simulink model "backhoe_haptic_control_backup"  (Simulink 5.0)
settings: Solver=ode5  StartTime=0.0  StopTime=inf  FixedStep=0.001  RelTol=1e-3
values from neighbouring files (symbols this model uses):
  a1 = 8.5    [startup.m]
  a2 = 48    [startup.m]
  a3 = 38+11/16    (= 38.6875)    [startup.m]
  a4 = 18.5    [startup.m]
  Butter_Order = 2    [startup.m]
  c1 = [-0.0009634 -0.4050766 2.3355377]    [startup.m]
  c2 = [ -0.00644514 2.23812750 22.79925627]    [startup.m]
  c3 = [-0.0057802 2.2376391 22.8266324]    [startup.m]
  c4 = [-0.0020828 1.5286223 20.3434998]    [startup.m]
  R1A = 10    [startup.m]
  R1B = 35.875    [startup.m]
  R2C = 36    [startup.m]
  R2D = 9+7/8    (= 9.875)    [startup.m]
  R3F = 4.5    [startup.m]
  R3G = 5.5    [startup.m]
  REF = 29.625    [startup.m]
  RFH = 9.5    [startup.m]
  RGH = 9.5    [startup.m]
  T01A = acos(RAJ/R1A)    [startup.m]
  T12C = acos((a2^2 + R2C^2 - R1C^2)/(2*a2*R2C))    [startup.m]
  T23D = 0.1317    [startup.m]
  TB12 = acos((R1B^2 + a2^2 - R2B^2)/(2*a2*R1B))    [startup.m]
  TD23 = acos((R2D^2 + a3^2 - R3D^2)/(2*a3*R2D))    [startup.m]
  TDFE = 0.0503    [startup.m]
  TG34 = 1.6966    [startup.m]
undefined symbols (not defined in the file or in its folder): channels, com, ended, Single, uint
libraries: dsparch4 x18, xpclib x8, simulink x1

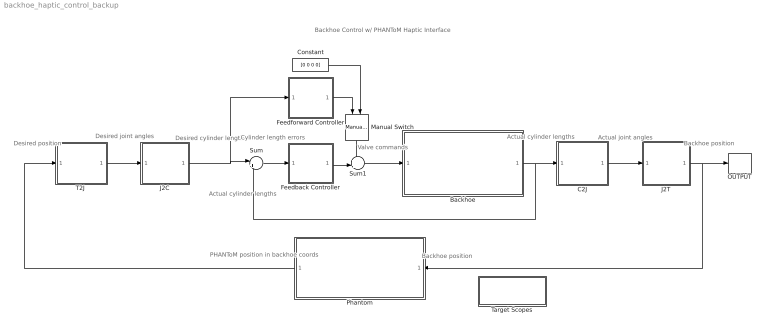
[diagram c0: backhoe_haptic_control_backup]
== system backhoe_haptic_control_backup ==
  note: Desired cylinder lengths
  note: Cylinder length errors
  note: Actual cylinder lengths
  note: Actual cylinder lengths
  note: Backhoe position
  note: Backhoe position
  note: PHANToM position in backhoe coords
  note: Desired joint angles
  note: Desired position
  note: Backhoe Control w/ PHANToM Haptic Interface
  note: Actual joint angles
  note: Valve commands
  Backhoe : Subsystem
  C2J : Subsystem
  Constant : Constant  Value=[0 0 0 0]
  Feedback Controller : Subsystem
  Feedforward Controller : Subsystem
  J2C : Subsystem
  J2T : Subsystem
  Manual Switch : simulink/Signal Routing/Manual Switch  Orientation=down  sw=0  action=0
  OUTPUT : ToWorkspace  VariableName=yb  SampleTime=-1  SaveFormat=StructureWithTime
  Phantom : Subsystem  Orientation=left
  Sum : Sum  Inputs=|+-
  Sum1 : Sum  Inputs=++|
  "T2J " : Subsystem
  Target Scopes : Subsystem
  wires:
  Sum/1 -> Feedback Controller/1(e)
  Backhoe/1(yc) -> Sum/2, C2J/1(yc)
  "T2J "/1(qdes) -> J2C/1(qdes)
  Feedback Controller/1(Us) -> Sum1/2
  Sum1/1 -> Backhoe/1(Us)
  Phantom/1(Yb_Desired) -> "T2J "/1(yp)
  J2C/1(ycdes) -> Sum/1, Feedforward Controller/1(ycdes)
  Manual Switch/1 -> Sum1/1
  Feedforward Controller/1(UsFF) -> Manual Switch/1
  Constant/1 -> Manual Switch/2
  C2J/1(q) -> J2T/1(q)
  J2T/1(yb) -> OUTPUT/1, Phantom/1(Yb)

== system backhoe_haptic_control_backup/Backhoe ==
  note: Valve commands
  note: Position sensor signals
  note: Cylinder lengths
  note: Pressure sensor signals
  Us : Inport
  Anti-Deadband Block : Subsystem
  Backhoe Interface : Subsystem
  Position sensor conversions : Subsystem
  T : Terminator
  yc : Outport
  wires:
  Backhoe Interface/1(Vpos) -> Position sensor conversions/1(Vc)
  Position sensor conversions/1(yc) -> yc/1
  Us/1 -> Anti-Deadband Block/1(us)
  Backhoe Interface/2(Vpres) -> T/1
  Anti-Deadband Block/1(Us) -> Backhoe Interface/1(Us)

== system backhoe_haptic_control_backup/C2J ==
  note: Swing
  note: q1
  note: Cylinder to Joint Transformation
  yc : Inport
  Boom : Subsystem
  Bucket : Subsystem
  Demux : Demux
  Mux : Mux
  Stick : Subsystem
  q : Outport
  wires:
  Mux/1 -> q/1, [GLOBAL_q]
  yc/1 -> Demux/1
  Boom/1(q2) -> Mux/2
  Demux/2 -> Boom/1(yc3)
  Demux/1 -> Mux/1
  Demux/3 -> Stick/1(yc4)
  Stick/1(q3) -> Mux/3
  Demux/4 -> Bucket/1(yc5)
  Bucket/1(q4) -> Mux/4

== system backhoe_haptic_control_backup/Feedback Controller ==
  e : Inport
  Demux : Demux
  Mux : Mux
  "boom [in/s] -> [V]" : Lookup  InputValues=[-1 0 1]  OutputValues=[-0.05 0 0.6]  ShowAdditionalParam=on
  "bucket [in/s] -> [V]" : Lookup  InputValues=[-1 0 1]  OutputValues=[-0.2 0 0.2]  ShowAdditionalParam=on
  "stick [in/s] -> [V]" : Lookup  InputValues=[-1 0 1]  OutputValues=[-0.2 0 0.2]  ShowAdditionalParam=on
  "swing [rad/s] -> [V]" : Lookup  InputValues=[-1 0 1]  OutputValues=[-0.2 0 0.2]  ShowAdditionalParam=on
  Us : Outport
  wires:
  e/1 -> [GLOBAL_e], Demux/1
  Demux/1 -> "swing [rad/s] -> [V]"/1
  "swing [rad/s] -> [V]"/1 -> Mux/1
  Demux/2 -> "boom [in/s] -> [V]"/1
  "boom [in/s] -> [V]"/1 -> Mux/2
  Demux/3 -> "stick [in/s] -> [V]"/1
  "stick [in/s] -> [V]"/1 -> Mux/3
  Demux/4 -> "bucket [in/s] -> [V]"/1
  "bucket [in/s] -> [V]"/1 -> Mux/4
  Mux/1 -> Us/1

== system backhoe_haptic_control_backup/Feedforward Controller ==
  note: This block uses empirical data from the open-loop velocity response to a constant voltage command to the valves. Relationships have been inverted to determine the required voltage to produce a desired velocity for each function.
  note: Feedforward Controller
  ycdes : Inport
  Demux : Demux
  Derivative : Derivative
  Filters : Subsystem
  Gain : Gain  Gain=1/3
  Mux : Mux
  "boom [in/s] -> [V]" : Lookup  InputValues=[-1.0 0 3.0]  OutputValues=[-0.25 0 0.25]  ShowAdditionalParam=on
  "bucket [in/s] -> [V]" : Lookup  InputValues=[-2.3 0 2.75]  OutputValues=[-0.25 0 0.25]  ShowAdditionalParam=on
  "stick [in/s] -> [V]" : Lookup  InputValues=[-1.6 0 1.75]  OutputValues=[-0.25 0 0.25]  ShowAdditionalParam=on
  "swing [rad/s] -> [V]" : Lookup  InputValues=[-0.6 0 0.7]  OutputValues=[-0.25 0 0.25]  ShowAdditionalParam=on
  UsFF : Outport
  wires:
  ycdes/1 -> Filters/1(unfiltered)
  Derivative/1 -> Demux/1
  Demux/1 -> "swing [rad/s] -> [V]"/1
  "swing [rad/s] -> [V]"/1 -> Mux/1
  Demux/2 -> "boom [in/s] -> [V]"/1
  "boom [in/s] -> [V]"/1 -> Mux/2
  Demux/3 -> "stick [in/s] -> [V]"/1
  "stick [in/s] -> [V]"/1 -> Mux/3
  Demux/4 -> "bucket [in/s] -> [V]"/1
  "bucket [in/s] -> [V]"/1 -> Mux/4
  Mux/1 -> Gain/1
  Filters/1(filtered) -> Derivative/1
  Gain/1 -> UsFF/1

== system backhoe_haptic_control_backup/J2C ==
  note: Joint Space -> Cylinder Space Transformation
  note: Swing Cylinders
  qdes : Inport
  Boom cylinder : Subsystem
  Bucket cylinder : Subsystem
  Demux : Demux
  Mux : Mux
  Stick cylinder : Subsystem
  overswing  protection : Saturate  UpperLimit=pi/3  LowerLimit=-pi/2
  ycdes : Outport
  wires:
  qdes/1 -> Demux/1
  Mux/1 -> ycdes/1
  Demux/2 -> Boom cylinder/1(q2)
  Boom cylinder/1(yc3) -> Mux/2
  Demux/3 -> Stick cylinder/1(q3)
  Stick cylinder/1(yc4) -> Mux/3
  Demux/4 -> Bucket cylinder/1(q4)
  Bucket cylinder/1(yc5) -> Mux/4
  Demux/1 -> overswing  protection/1
  overswing  protection/1 -> Mux/1

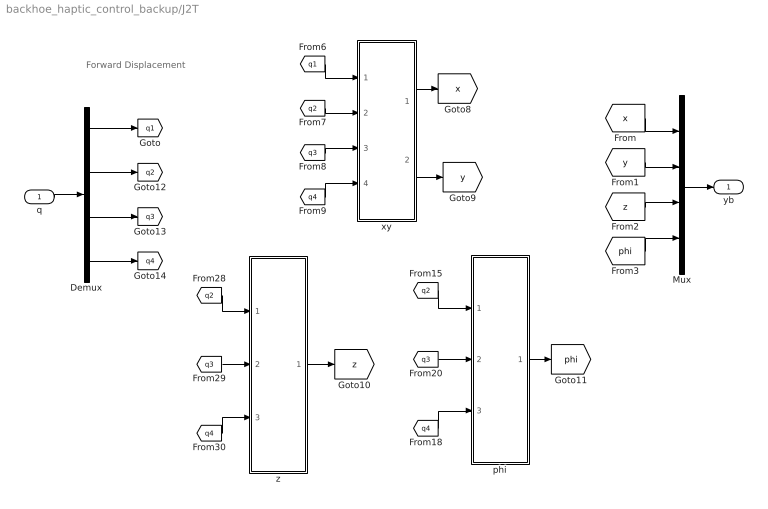
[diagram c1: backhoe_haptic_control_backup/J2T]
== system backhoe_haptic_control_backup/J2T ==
  note: Forward Displacement
  q : Inport
  Demux : Demux
  Mux : Mux
  phi : Subsystem
  xy : Subsystem
  z : Subsystem
  yb : Outport
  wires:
  [q2] -> z/1(q2)
  [q3] -> z/2(q3)
  [q4] -> z/3(q4)
  z/1(z) -> [z]
  q/1 -> Demux/1
  Demux/2 -> [q2]
  Demux/1 -> [q1]
  Demux/3 -> [q3]
  Demux/4 -> [q4]
  [q2] -> phi/1(q2)
  [q3] -> phi/2(q3)
  phi/1(phi) -> [phi]
  Mux/1 -> yb/1
  [x] -> Mux/1
  [y] -> Mux/2
  [z] -> Mux/3
  [phi] -> Mux/4
  xy/1(x) -> [x]
  [q1] -> xy/1(q1)
  [q2] -> xy/2(q2)
  [q3] -> xy/3(q3)
  [q4] -> xy/4(q4)
  [q4] -> phi/3(q4)
  xy/2(y) -> [y]

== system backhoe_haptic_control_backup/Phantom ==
  Yb : Inport
  Phantom Interface : Subsystem
  Supervisory Control : Subsystem
  Yb_Desired : Outport
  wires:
  Yb/1 -> Supervisory Control/1(Y_Bh)
  Supervisory Control/1(Y_Bh_ref) -> Yb_Desired/1, [GLOBAL_YB_DES]
  Phantom Interface/2(Ph_Time) -> Supervisory Control/3(Ph_Time)
  Phantom Interface/3(Ph_Flag) -> Supervisory Control/4(Ph Flag)
  Supervisory Control/3(OUt_Flag) -> Phantom Interface/2(Bh_Flag)
  Supervisory Control/2(Send2Ph) -> Phantom Interface/1(Yb)
  Phantom Interface/1("Yp ") -> Supervisory Control/2(Y_Ph_In)

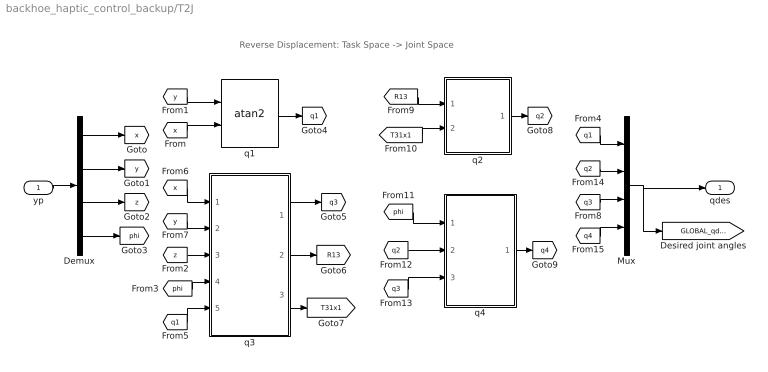
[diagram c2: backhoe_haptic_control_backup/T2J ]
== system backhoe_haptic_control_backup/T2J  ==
  note: Reverse Displacement: Task Space -> Joint Space
  yp : Inport
  Demux : Demux
  Mux : Mux
  q1 : Trigonometry  Operator=atan2
  q2 : Subsystem
  q3 : Subsystem
  q4 : Subsystem
  qdes : Outport
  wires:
  [x] -> q3/1(x)
  [y] -> q3/2(y)
  [z] -> q3/3(z)
  [phi] -> q3/4(phi)
  [q1] -> q3/5(q1)
  q3/1(q3) -> [q3]
  q3/2(R13) -> [R13]
  [y] -> q1/1
  [x] -> q1/2
  q1/1 -> [q1]
  q3/3(T31x1) -> [T31x1]
  [R13] -> q2/1(R13)
  [T31x1] -> q2/2(T31x1)
  [q3] -> q4/3(q3)
  [q2] -> q4/2(q2)
  [phi] -> q4/1(phi)
  q2/1(q2) -> [q2]
  q4/1(q4) -> [q4]
  Mux/1 -> qdes/1, [GLOBAL_qdes]
  [q1] -> Mux/1
  [q3] -> Mux/3
  [q2] -> Mux/2
  [q4] -> Mux/4
  yp/1 -> Demux/1
  Demux/1 -> [x]
  Demux/2 -> [y]
  Demux/3 -> [z]
  Demux/4 -> [phi]

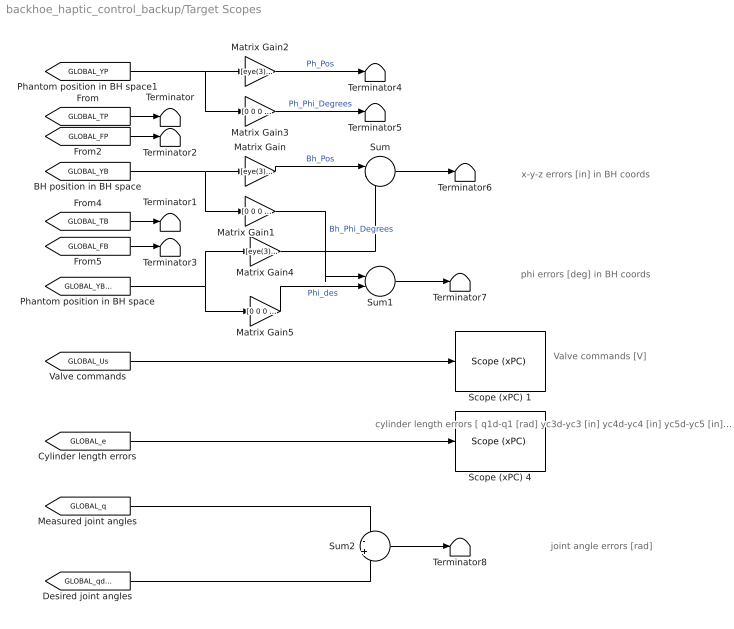
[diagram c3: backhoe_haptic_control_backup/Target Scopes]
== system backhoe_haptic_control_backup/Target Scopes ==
  note: x-y-z errors [in] in BH coords
  note: phi errors [deg] in BH coords
  note: Valve commands [V]
  note: cylinder length errors [ q1d-q1 [rad] yc3d-yc3 [in] yc4d-yc4 [in] yc5d-yc5 [in] ]
  note: joint angle errors [rad]
  Matrix Gain : Gain  Gain=[eye(3) zeros(3,1)]  Multiplication=Matrix(K*u)
  Matrix Gain1 : Gain  Gain=[0 0 0 180/pi]  Multiplication=Matrix(K*u)
  Matrix Gain2 : Gain  Gain=[eye(3) zeros(3,1)]  Multiplication=Matrix(K*u)
  Matrix Gain3 : Gain  Gain=[0 0 0 180/pi]  Multiplication=Matrix(K*u)
  Matrix Gain4 : Gain  Gain=[eye(3) zeros(3,1)]  Multiplication=Matrix(K*u)
  Matrix Gain5 : Gain  Gain=[0 0 0 180/pi]  Multiplication=Matrix(K*u)
  Scope (xPC) 1 : xpclib/Misc./Scope (xPC)   scopeno=3  scopetype=Target  viewmode=Graphical redraw  grid=on  ylimits=[0,12]  autostart=on  nosamples=1000  noprepostsamples=0  interleave=1  triggermode=FreeRun  triggersignal=1  triggerlevel=0.0  triggerslope=either  triggerscope=1  triggersample=0
  Scope (xPC) 4 : xpclib/Misc./Scope (xPC)   scopeno=4  scopetype=Target  viewmode=Graphical redraw  grid=on  ylimits=[-5,5]  autostart=on  nosamples=1000  noprepostsamples=0  interleave=1  triggermode=FreeRun  triggersignal=1  triggerlevel=0.0  triggerslope=either  triggerscope=1  triggersample=0
  Sum : Sum  Inputs=|-+
  Sum1 : Sum  Inputs=|-+
  Sum2 : Sum  Inputs=-+
  Terminator{,1..8} (9 alike) : Terminator
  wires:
  [GLOBAL_TP] -> Terminator/1
  [GLOBAL_TB] -> Terminator1/1
  [GLOBAL_YB] -> Matrix Gain/1, Matrix Gain1/1
  [GLOBAL_YP] -> Matrix Gain2/1, Matrix Gain3/1
  [GLOBAL_FP] -> Terminator2/1
  [GLOBAL_FB] -> Terminator3/1
  Sum1/1 -> Terminator7/1
  Matrix Gain5/1 -> Sum1/2  "Phi_des"
  Matrix Gain1/1 -> Sum1/1  "Bh_Phi_Degrees"
  Sum/1 -> Terminator6/1
  Matrix Gain/1 -> Sum/1  "Bh_Pos"
  Matrix Gain4/1 -> Sum/2
  Matrix Gain2/1 -> Terminator4/1  "Ph_Pos"
  Matrix Gain3/1 -> Terminator5/1  "Ph_Phi_Degrees"
  [GLOBAL_Us] -> Scope (xPC) 1/1
  Sum2/1 -> Terminator8/1
  [GLOBAL_YB_DES] -> Matrix Gain4/1, Matrix Gain5/1
  [GLOBAL_e] -> Scope (xPC) 4/1
  [GLOBAL_q] -> Sum2/1
  [GLOBAL_qdes] -> Sum2/2

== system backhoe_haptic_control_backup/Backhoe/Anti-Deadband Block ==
  note: This block take a servo commmand that saturates at +-1 and converts it into valve signals. "u" in the input signal which a 4-vector. Neutral is half the voltage supplied Vc to the valves which should 6V = 1/2 * 12V. Commands to the valve must be between 25% AND 75% of Vc where 50% is neutral or the "zero command" that tell the valve to stop flow to the valve. Neutral can either be set at 6V of measure from Channel 15.
  us : Inport
  Demux : Demux
  Look-Up Table{,1..3} (4 alike) : Lookup  InputValues=[-1 -0.02 0.02 1]  OutputValues=[3 5.45 6.55 9]  ShowAdditionalParam=on  LookUpMeth=Interpolation-Use End Values  OutDataTypeMode=double
  Mux : Mux
  Us : Outport
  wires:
  Look-Up Table/1 -> Mux/1
  Look-Up Table1/1 -> Mux/2
  Demux/1 -> Look-Up Table/1
  Demux/2 -> Look-Up Table1/1
  Demux/3 -> Look-Up Table2/1
  Look-Up Table2/1 -> Mux/3
  Demux/4 -> Look-Up Table3/1
  Look-Up Table3/1 -> Mux/4
  Mux/1 -> Us/1
  us/1 -> Demux/1

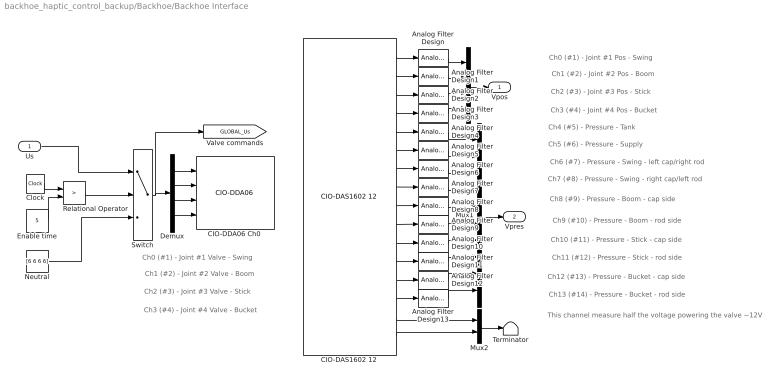
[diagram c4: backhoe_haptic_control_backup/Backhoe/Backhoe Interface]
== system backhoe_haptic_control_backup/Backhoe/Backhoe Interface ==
  note: Ch0 (#1) - Joint #1 Valve - Swing
  note: Ch1 (#2) - Joint #2 Valve - Boom
  note: Ch2 (#3) - Joint #3 Valve - Stick
  note: Ch3 (#4) - Joint #4 Valve - Bucket
  note: Ch0 (#1) - Joint #1 Pos - Swing
  note: Ch1 (#2) - Joint #2 Pos - Boom
  note: Ch2 (#3) - Joint #3 Pos - Stick
  note: Ch3 (#4) - Joint #4 Pos - Bucket
  note: Ch4 (#5) - Pressure - Tank
  note: Ch5 (#6) - Pressure - Supply
  note: Ch6 (#7) - Pressure - Swing - left cap/right rod
  note: Ch7 (#8) - Pressure - Swing - right cap/left rod
  note: Ch8 (#9) - Pressure - Boom - cap side
  note: Ch9 (#10) - Pressure - Boom - rod side
  note: Ch10 (#11) - Pressure - Stick - cap side
  note: Ch11 (#12) - Pressure - Stick - rod side
  note: Ch12 (#13) - Pressure - Bucket - cap side
  note: Ch13 (#14) - Pressure - Bucket - rod side
  note: This channel measure half the voltage powering the valve ~12V
  Us : Inport
  Analog Filter Design{,1..13} (14 alike) : dsparch4/Analog Filter Design  method=Butterworth  filttype=Lowpass  N=Butter_Order  Wlo=Butter_Rad  Whi=80  Rp=2  Rs=40
  "CIO-DAS1602 12 " : xpclib/A//D/Computer Boards/CIO-DAS1602 12   channel=16  range=0-10V  mux=Single-ended (16 channels)  sampletime=0.001  baseaddress=0x340
  "CIO-DDA06 Ch0 " : xpclib/D//A/Computer Boards/CIO-DDA06   channel=[1 2 3 4]  range=[10 10 10 10]  reset=[1 1 1 1]  initValue=[6 6 6 6]  sampletime=0.001  baseaddress=0x300
  Clock : Clock
  Demux : Demux
  Enable time : Constant  Value=5
  Mux : Mux
  Mux1 : Mux  Inputs=10
  Mux2 : Mux  Inputs=2
  Neutral : Constant  Value=[6 6 6 6]  ShowAdditionalParam=on
  Relational Operator : RelationalOperator  Operator=>  ShowAdditionalParam=on
  Switch : Switch  Threshold=0.5  ShowAdditionalParam=on
  Terminator : Terminator
  Vpos : Outport
  Vpres : Outport  Port=2
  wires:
  Demux/1 -> "CIO-DDA06 Ch0 "/1
  Demux/2 -> "CIO-DDA06 Ch0 "/2
  Demux/3 -> "CIO-DDA06 Ch0 "/3
  Demux/4 -> "CIO-DDA06 Ch0 "/4
  Mux/1 -> Vpos/1
  "CIO-DAS1602 12 "/1 -> Analog Filter Design/1
  Analog Filter Design/1 -> Mux/1
  "CIO-DAS1602 12 "/2 -> Analog Filter Design1/1
  "CIO-DAS1602 12 "/3 -> Analog Filter Design2/1
  "CIO-DAS1602 12 "/4 -> Analog Filter Design3/1
  Analog Filter Design1/1 -> Mux/2
  Analog Filter Design2/1 -> Mux/3
  Analog Filter Design3/1 -> Mux/4
  "CIO-DAS1602 12 "/5 -> Analog Filter Design4/1
  "CIO-DAS1602 12 "/6 -> Analog Filter Design5/1
  "CIO-DAS1602 12 "/7 -> Analog Filter Design6/1
  "CIO-DAS1602 12 "/8 -> Analog Filter Design7/1
  "CIO-DAS1602 12 "/9 -> Analog Filter Design8/1
  "CIO-DAS1602 12 "/10 -> Analog Filter Design9/1
  "CIO-DAS1602 12 "/11 -> Analog Filter Design10/1
  "CIO-DAS1602 12 "/12 -> Analog Filter Design11/1
  "CIO-DAS1602 12 "/13 -> Analog Filter Design12/1
  "CIO-DAS1602 12 "/14 -> Analog Filter Design13/1
  "CIO-DAS1602 12 "/15 -> Mux2/1
  Analog Filter Design4/1 -> Mux1/1
  Analog Filter Design5/1 -> Mux1/2
  Analog Filter Design6/1 -> Mux1/3
  Analog Filter Design7/1 -> Mux1/4
  Analog Filter Design8/1 -> Mux1/5
  Analog Filter Design9/1 -> Mux1/6
  Analog Filter Design10/1 -> Mux1/7
  Analog Filter Design11/1 -> Mux1/8
  Analog Filter Design12/1 -> Mux1/9
  Analog Filter Design13/1 -> Mux1/10
  Mux1/1 -> Vpres/1
  Mux2/1 -> Terminator/1
  "CIO-DAS1602 12 "/16 -> Mux2/2
  Switch/1 -> Demux/1, [GLOBAL_Us]
  Clock/1 -> Relational Operator/1
  Enable time/1 -> Relational Operator/2
  Relational Operator/1 -> Switch/2
  Neutral/1 -> Switch/3
  Us/1 -> Switch/1

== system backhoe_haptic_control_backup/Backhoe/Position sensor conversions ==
  note: Sensor Conversions
  Vc : Inport
  Boom sensor : Subsystem
  Bucket sensor : Subsystem
  Demux : Demux
  Mux : Mux
  Stick sensor : Subsystem
  Swing pot : Subsystem
  yc : Outport
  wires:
  Vc/1 -> Demux/1
  Demux/1 -> Swing pot/1(Vc1)
  Demux/2 -> Boom sensor/1(Vc2)
  Swing pot/1(q1) -> Mux/1
  Boom sensor/1(yc3) -> Mux/2
  Demux/3 -> Stick sensor/1(Vc3)
  Stick sensor/1(yc4) -> Mux/3
  Mux/1 -> yc/1
  Demux/4 -> Bucket sensor/1(Vc4)
  Bucket sensor/1(yc5) -> Mux/4

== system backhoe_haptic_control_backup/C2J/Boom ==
  note: TA1B
  yc3 : Inport
  CosineLawA : Subsystem
  R1A : Constant  Value=R1A
  R1B : Constant  Value=R1B
  Sum : Sum  Inputs=+---
  T01A : Constant  Value=T01A
  TA1B : Constant  Value=TB12
  pi : Constant  Value=pi
  q2 : Outport
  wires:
  pi/1 -> Sum/1
  T01A/1 -> Sum/2
  TA1B/1 -> Sum/4
  CosineLawA/1(theta) -> Sum/3
  R1A/1 -> CosineLawA/1(r1)
  R1B/1 -> CosineLawA/2(r2)
  Sum/1 -> q2/1
  yc3/1 -> CosineLawA/3(r3)

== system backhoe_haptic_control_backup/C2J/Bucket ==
  yc5 : Inport
  R3F : Constant  Value=R3F
  R3G : Constant  Value=R3G
  R3H : Subsystem
  REF : Constant  Value=REF
  RFH : Constant  Value=RFH
  RGH : Constant  Value=RGH
  Sum : Sum  Inputs=+----
  T23D : Constant  Value=T23D
  TEFH : Subsystem
  TF3H : Subsystem
  TG34 : Constant  Value=TG34
  TH3G : Subsystem
  THF3 : Subsystem
  pi : Constant  Value=3*pi
  q4 : Outport
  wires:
  TEFH/1(TEFH) -> THF3/1(TEFH)
  REF/1 -> TEFH/1(r1)
  yc5/1 -> TEFH/3(r3)
  RFH/1 -> TEFH/2(r2), R3H/2(RFH), TF3H/3(r3)
  THF3/1(THF3) -> R3H/1(THF3)
  R3F/1 -> TF3H/1(r1)
  R3H/1(R3H) -> TF3H/2(r2), TH3G/1(r1)
  R3G/1 -> TH3G/2(r2)
  RGH/1 -> TH3G/3(r3)
  pi/1 -> Sum/1
  Sum/1 -> q4/1
  T23D/1 -> Sum/5
  TG34/1 -> Sum/4
  TH3G/1(TH3G) -> Sum/2
  TF3H/1(TF3H) -> Sum/3

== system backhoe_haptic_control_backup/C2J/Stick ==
  note: TC2D
  yc4 : Inport
  CosineLawA : Subsystem
  R2C : Constant  Value=R2C
  R2D : Constant  Value=R2D
  Sum : Sum  Inputs=+---
  T12C : Constant  Value=T12C
  TD23 : Constant  Value=TD23
  pi : Constant  Value=3*pi
  q3 : Outport
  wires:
  pi/1 -> Sum/1
  T12C/1 -> Sum/2
  TD23/1 -> Sum/4
  CosineLawA/1(theta) -> Sum/3
  R2C/1 -> CosineLawA/1(r1)
  R2D/1 -> CosineLawA/2(r2)
  Sum/1 -> q3/1
  yc4/1 -> CosineLawA/3(r3)

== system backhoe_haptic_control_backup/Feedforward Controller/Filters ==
  unfiltered : Inport
  Analog Filter Design{,1..3} (4 alike) : dsparch4/Analog Filter Design  method=Butterworth  filttype=Lowpass  N=2  Wlo=2*pi*5  Whi=80  Rp=2  Rs=40
  Demux : Demux
  Mux : Mux
  filtered : Outport
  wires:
  unfiltered/1 -> Demux/1
  Demux/1 -> Analog Filter Design/1
  Analog Filter Design/1 -> Mux/1
  Demux/2 -> Analog Filter Design1/1
  Analog Filter Design1/1 -> Mux/2
  Demux/3 -> Analog Filter Design2/1
  Analog Filter Design2/1 -> Mux/3
  Demux/4 -> Analog Filter Design3/1
  Analog Filter Design3/1 -> Mux/4
  Mux/1 -> filtered/1

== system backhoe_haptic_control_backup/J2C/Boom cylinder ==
  q2 : Inport
  Constant : Constant  Value=pi
  Constant1 : Constant  Value=T01A
  Constant2 : Constant  Value=TB12
  CosineLawB : Subsystem
  Sum : Sum  Inputs=+---
  yc3 : Outport
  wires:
  Constant/1 -> Sum/1
  Constant1/1 -> Sum/2
  Sum/1 -> CosineLawB/1(TA1B)
  CosineLawB/1(yc3) -> yc3/1
  q2/1 -> Sum/3
  Constant2/1 -> Sum/4

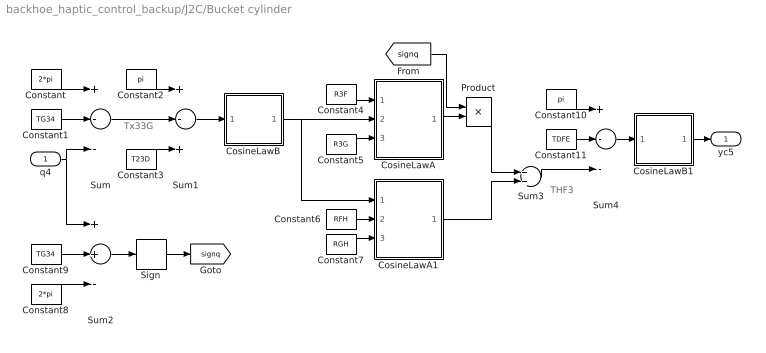
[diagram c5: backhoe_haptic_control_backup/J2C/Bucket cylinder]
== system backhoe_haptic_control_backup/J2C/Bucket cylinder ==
  note: Tx33G
  note: THF3
  q4 : Inport
  Constant : Constant  Value=2*pi
  Constant1 : Constant  Value=TG34
  Constant10 : Constant  Value=pi
  Constant11 : Constant  Value=TDFE
  Constant2 : Constant  Value=pi
  Constant3 : Constant  Value=T23D
  Constant4 : Constant  Value=R3F
  Constant5 : Constant  Value=R3G
  Constant6 : Constant  Value=RFH
  Constant7 : Constant  Value=RGH
  Constant8 : Constant  Value=2*pi
  Constant9 : Constant  Value=TG34
  CosineLawA : Subsystem
  CosineLawA1 : Subsystem
  CosineLawB : Subsystem
  CosineLawB1 : Subsystem
  Product : Product
  Sign : Signum
  Sum : Sum  Inputs=+--
  Sum1 : Sum  Inputs=+-+
  Sum2 : Sum  Inputs=++-
  Sum3 : Sum
  Sum4 : Sum  Inputs=+--
  yc5 : Outport
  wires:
  Constant/1 -> Sum/1
  Constant1/1 -> Sum/2
  Sum/1 -> Sum1/2
  Constant2/1 -> Sum1/1
  Constant3/1 -> Sum1/3
  Sum1/1 -> CosineLawB/1(TG3F)
  CosineLawB/1(rFG) -> CosineLawA/2(r2), CosineLawA1/1(r1)
  Constant4/1 -> CosineLawA/1(r1)
  Constant5/1 -> CosineLawA/3(r3)
  Constant6/1 -> CosineLawA1/2(r2)
  Constant7/1 -> CosineLawA1/3(r3)
  Constant9/1 -> Sum2/2
  Constant8/1 -> Sum2/3
  Sum2/1 -> Sign/1
  [signq] -> Product/1
  CosineLawA/1(T3FG) -> Product/2
  Sign/1 -> [signq]
  Product/1 -> Sum3/1
  CosineLawA1/1(THFG) -> Sum3/2
  Constant10/1 -> Sum4/1
  Sum3/1 -> Sum4/3
  Constant11/1 -> Sum4/2
  Sum4/1 -> CosineLawB1/1(TEFH)
  CosineLawB1/1(yc5) -> yc5/1
  q4/1 -> Sum/3, Sum2/1

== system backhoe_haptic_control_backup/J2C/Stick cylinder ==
  q3 : Inport
  Constant : Constant  Value=pi
  Constant1 : Constant  Value=TD23
  Constant2 : Constant  Value=T12C
  CosineLawB : Subsystem
  Sum : Sum  Inputs=+---
  yc4 : Outport
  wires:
  Constant/1 -> Sum/1
  Constant1/1 -> Sum/2
  Sum/1 -> CosineLawB/1(TC2D)
  CosineLawB/1(yc4) -> yc4/1
  q3/1 -> Sum/3
  Constant2/1 -> Sum/4

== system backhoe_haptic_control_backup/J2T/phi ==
  q2 : Inport
  q3 : Inport  Port=2
  q4 : Inport  Port=3
  Constant : Constant  Value=3*pi
  Sum : Sum  Inputs=+++-
  phi : Outport
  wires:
  q2/1 -> Sum/1
  q3/1 -> Sum/2
  q4/1 -> Sum/3
  Constant/1 -> Sum/4
  Sum/1 -> phi/1

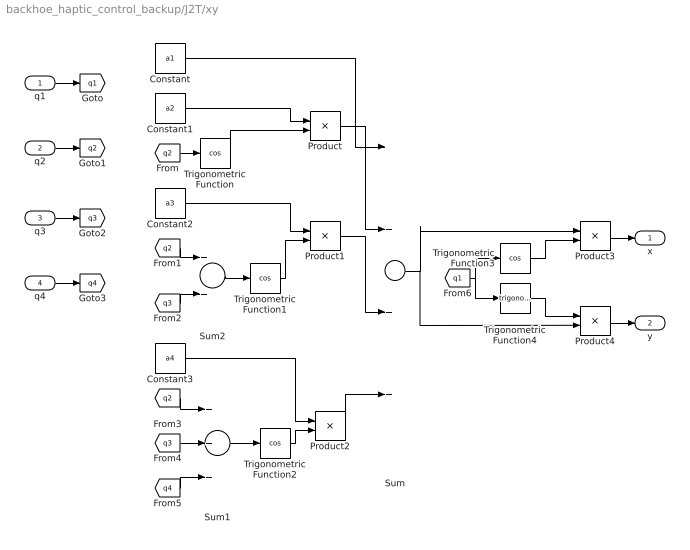
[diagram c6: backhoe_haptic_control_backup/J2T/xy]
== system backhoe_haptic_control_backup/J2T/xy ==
  q1 : Inport
  q2 : Inport  Port=2
  q3 : Inport  Port=3
  q4 : Inport  Port=4
  Constant : Constant  Value=a1
  Constant1 : Constant  Value=a2
  Constant2 : Constant  Value=a3
  Constant3 : Constant  Value=a4
  Product{,1..4} (5 alike) : Product
  Sum : Sum  Inputs=++++
  Sum1 : Sum  Inputs=+++
  Sum2 : Sum
  Trigonometric Function{,1..3} (4 alike) : Trigonometry  Operator=cos
  Trigonometric Function4 : Trigonometry
  x : Outport
  y : Outport  Port=2
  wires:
  q1/1 -> [q1]
  q2/1 -> [q2]
  q3/1 -> [q3]
  q4/1 -> [q4]
  Constant/1 -> Sum/1
  Product/1 -> Sum/2
  Constant1/1 -> Product/1
  [q3] -> Sum2/2
  [q2] -> Sum2/1
  Constant2/1 -> Product1/1
  Product1/1 -> Sum/3
  Product2/1 -> Sum/4
  Constant3/1 -> Product2/1
  [q2] -> Sum1/1
  [q3] -> Sum1/2
  [q4] -> Sum1/3
  Product3/1 -> x/1
  Sum/1 -> Product4/2, Product3/1
  Trigonometric Function/1 -> Product/2
  [q2] -> Trigonometric Function/1
  Sum2/1 -> Trigonometric Function1/1
  Trigonometric Function1/1 -> Product1/2
  Sum1/1 -> Trigonometric Function2/1
  Trigonometric Function2/1 -> Product2/2
  Product4/1 -> y/1
  Trigonometric Function3/1 -> Product3/2
  [q1] -> Trigonometric Function3/1, Trigonometric Function4/1
  Trigonometric Function4/1 -> Product4/1

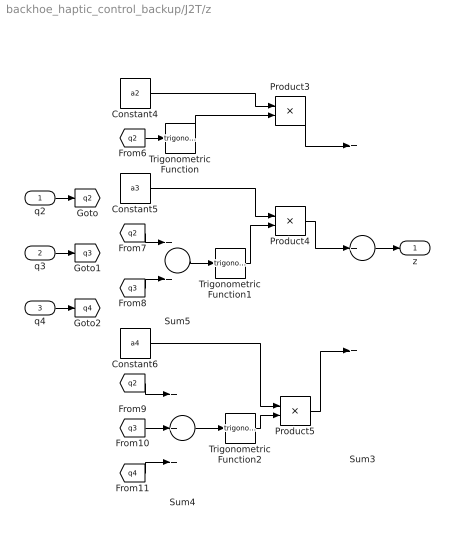
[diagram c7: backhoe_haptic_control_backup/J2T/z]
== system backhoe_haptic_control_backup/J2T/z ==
  q2 : Inport
  q3 : Inport  Port=2
  q4 : Inport  Port=3
  Constant4 : Constant  Value=a2
  Constant5 : Constant  Value=a3
  Constant6 : Constant  Value=a4
  Product3 : Product
  Product4 : Product
  Product5 : Product
  Sum3 : Sum  Inputs=+++
  Sum4 : Sum  Inputs=+++
  Sum5 : Sum
  Trigonometric Function : Trigonometry
  Trigonometric Function1 : Trigonometry
  Trigonometric Function2 : Trigonometry
  z : Outport
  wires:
  q3/1 -> [q3]
  q4/1 -> [q4]
  q2/1 -> [q2]
  Constant4/1 -> Product3/1
  [q3] -> Sum5/2
  [q2] -> Sum5/1
  Constant5/1 -> Product4/1
  Constant6/1 -> Product5/1
  [q2] -> Sum4/1
  [q3] -> Sum4/2
  [q4] -> Sum4/3
  Trigonometric Function/1 -> Product3/2
  [q2] -> Trigonometric Function/1
  Sum5/1 -> Trigonometric Function1/1
  Trigonometric Function1/1 -> Product4/2
  Sum4/1 -> Trigonometric Function2/1
  Trigonometric Function2/1 -> Product5/2
  Product3/1 -> Sum3/1
  Product4/1 -> Sum3/2
  Product5/1 -> Sum3/3
  Sum3/1 -> z/1

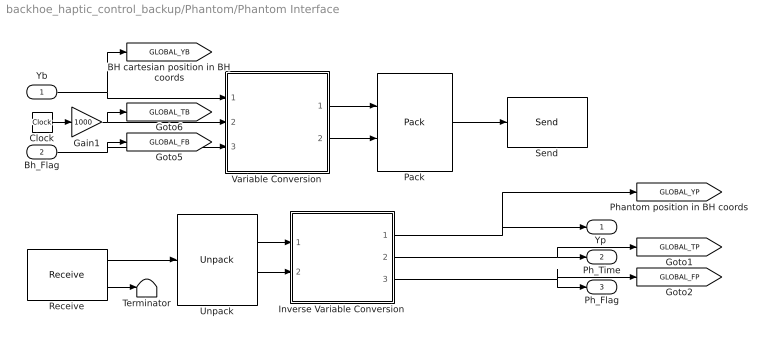
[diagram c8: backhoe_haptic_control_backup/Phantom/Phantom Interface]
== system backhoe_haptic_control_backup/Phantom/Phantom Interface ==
  Yb : Inport
  Bh_Flag : Inport  Port=2
  Clock : Clock
  Gain1 : Gain  Gain=1000  ShowAdditionalParam=on  OutDataTypeMode=Specify via dialog  OutDataType=uint(32)
  Inverse Variable Conversion : Subsystem
  Pack : xpclib/UDP/Pack  datatypes={'double','uint32'}  byteAlign=8
  Receive : xpclib/UDP/Receive  ipAddress=0.0.0.0  ipPort=com.Ph2Bh_Port  width=com.Ph2Bh_Bytes  sampletime=Sampling_Time
  Send : xpclib/UDP/Send  ipAddress=com.SendIP  ipPort=com.Bh2Ph_Port  sampletime=Sampling_Time
  Terminator : Terminator
  Unpack : xpclib/UDP/Unpack  dimensions=com.Ph2Bh_Port_Dim  datatypes={'double','uint32'}  byteAlign=8
  Variable Conversion : Subsystem
  "Yp " : Outport
  Ph_Time : Outport  Port=2
  Ph_Flag : Outport  Port=3
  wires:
  Receive/2 -> Terminator/1
  Receive/1 -> Unpack/1
  Pack/1 -> Send/1
  Yb/1 -> Variable Conversion/1(Yb), [GLOBAL_YB]
  Bh_Flag/1 -> [GLOBAL_FB], Variable Conversion/3(Bh_Flag)
  Unpack/1 -> Inverse Variable Conversion/1(doubles)
  Inverse Variable Conversion/3(Ph_Flag) -> Ph_Flag/1, [GLOBAL_FP]
  Inverse Variable Conversion/2(Ph_Time) -> Ph_Time/1, [GLOBAL_TP]
  Unpack/2 -> Inverse Variable Conversion/2(uint32s)
  Variable Conversion/2(uint32s) -> Pack/2
  Variable Conversion/1(doubles) -> Pack/1
  Clock/1 -> Gain1/1
  Gain1/1 -> [GLOBAL_TB], Variable Conversion/2(Bh_Time)
  Inverse Variable Conversion/1(Yp) -> "Yp "/1, [GLOBAL_YP]

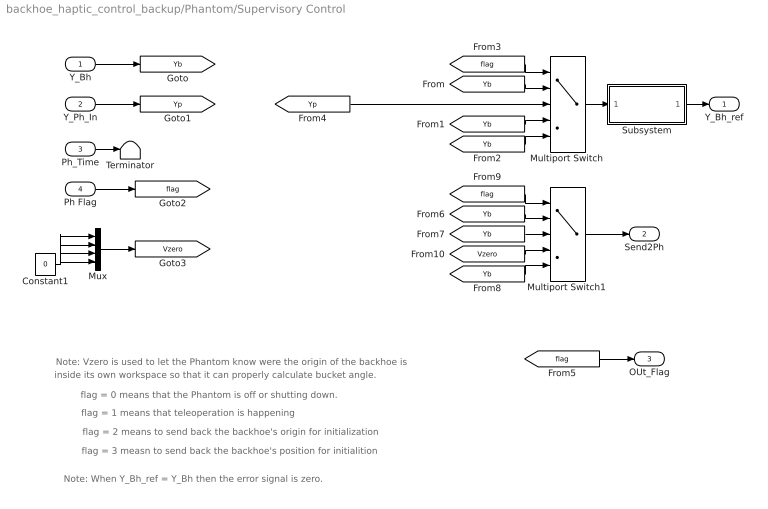
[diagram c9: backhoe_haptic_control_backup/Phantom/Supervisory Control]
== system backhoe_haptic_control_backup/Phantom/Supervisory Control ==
  note: Note: Vzero is used to let the Phantom know were the origin of the backhoe is
  note: flag = 0 means that the Phantom is off or shutting down.
  note: flag = 3 measn to send back the backhoe's position for initialition
  note: inside its own workspace so that it can properly calculate bucket angle.
  note: flag = 1 means that teleoperation is happening
  note: flag = 2 means to send back the backhoe's origin for initialization
  note: Note: When Y_Bh_ref = Y_Bh then the error signal is zero.
  Y_Bh : Inport
  Y_Ph_In : Inport  Port=2
  Ph_Time : Inport  Port=3
  Ph Flag : Inport  Port=4
  Constant1 : Constant  Value=0
  Multiport Switch : MultiPortSwitch  ShowAdditionalParam=on  zeroidx=on
  Multiport Switch1 : MultiPortSwitch  ShowAdditionalParam=on  zeroidx=on
  Mux : Mux
  Subsystem : Subsystem
  Terminator : Terminator
  Y_Bh_ref : Outport
  Send2Ph : Outport  Port=2
  OUt_Flag : Outport  Port=3
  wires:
  Ph_Time/1 -> Terminator/1
  [flag] -> OUt_Flag/1
  Y_Bh/1 -> [Yb]
  Ph Flag/1 -> [flag]
  Constant1/1 -> Mux/1, Mux/4, Mux/3, Mux/2
  Mux/1 -> [Vzero]
  [Yb] -> Multiport Switch/2
  [Yb] -> Multiport Switch/4
  [Yb] -> Multiport Switch/5
  [flag] -> Multiport Switch/1
  [Yb] -> Multiport Switch1/2
  [Vzero] -> Multiport Switch1/4
  [Yb] -> Multiport Switch1/5
  [flag] -> Multiport Switch1/1
  [Yb] -> Multiport Switch1/3
  Multiport Switch1/1 -> Send2Ph/1
  Multiport Switch/1 -> Subsystem/1(Yp)
  Subsystem/1(Y_Bh_REF) -> Y_Bh_ref/1
  [Yp] -> Multiport Switch/3
  Y_Ph_In/1 -> [Yp]

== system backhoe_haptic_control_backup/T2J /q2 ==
  note: T213
  R13 : Inport
  T31x1 : Inport  Port=2
  CosineLawA : Subsystem
  Sum : Sum  Inputs=|++
  a2 : Constant  Value=a2
  a3 : Constant  Value=a3
  q2 : Outport
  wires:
  a2/1 -> CosineLawA/1(r1)
  a3/1 -> CosineLawA/3(r3)
  CosineLawA/1(theta) -> Sum/1
  Sum/1 -> q2/1
  R13/1 -> CosineLawA/2(r2)
  T31x1/1 -> Sum/2

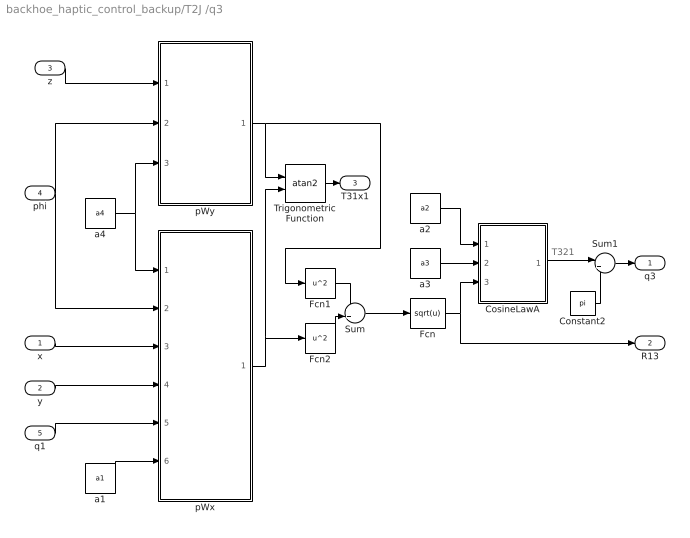
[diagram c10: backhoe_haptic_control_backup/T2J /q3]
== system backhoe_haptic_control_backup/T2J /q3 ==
  note: T321
  x : Inport
  y : Inport  Port=2
  z : Inport  Port=3
  phi : Inport  Port=4
  q1 : Inport  Port=5
  Constant2 : Constant  Value=pi
  CosineLawA : Subsystem
  Fcn : Fcn  Expr=sqrt(u)
  Fcn1 : Fcn  Expr=u^2
  Fcn2 : Fcn  Expr=u^2
  Sum : Sum
  Sum1 : Sum  Inputs=|++
  Trigonometric Function : Trigonometry  Operator=atan2
  a1 : Constant  Value=a1
  a2 : Constant  Value=a2
  a3 : Constant  Value=a3
  a4 : Constant  Value=a4
  pWx : Subsystem
  pWy : Subsystem
  q3 : Outport
  R13 : Outport  Port=2
  T31x1 : Outport  Port=3
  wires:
  a1/1 -> pWx/6(a1)
  q1/1 -> pWx/5(q1)
  y/1 -> pWx/4(y)
  x/1 -> pWx/3(x)
  a4/1 -> pWx/1(a4), pWy/3(a4)
  z/1 -> pWy/1(z)
  phi/1 -> pWx/2(phi), pWy/2(phi)
  pWy/1(pWy) -> Fcn1/1, Trigonometric Function/1
  Trigonometric Function/1 -> T31x1/1
  Fcn1/1 -> Sum/1
  Fcn2/1 -> Sum/2
  Sum/1 -> Fcn/1
  pWx/1(pWx) -> Fcn2/1, Trigonometric Function/2
  a3/1 -> CosineLawA/2(r2)
  a2/1 -> CosineLawA/1(r1)
  Fcn/1 -> CosineLawA/3(r3), R13/1
  Sum1/1 -> q3/1
  Constant2/1 -> Sum1/2
  CosineLawA/1(theta) -> Sum1/1

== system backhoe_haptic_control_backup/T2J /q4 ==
  phi : Inport
  q2 : Inport  Port=2
  q3 : Inport  Port=3
  Constant : Constant  Value=3*pi
  Sum : Sum  Inputs=+--+
  q4 : Outport
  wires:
  phi/1 -> Sum/1
  q2/1 -> Sum/2
  Sum/1 -> q4/1
  q3/1 -> Sum/3
  Constant/1 -> Sum/4

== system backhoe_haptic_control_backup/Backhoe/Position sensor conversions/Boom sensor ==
  Vc2 : Inport
  Fcn : Fcn  Expr=u^2
  Product : Product
  Product1 : Product
  Sum : Sum  Inputs=+++
  c10 : Constant  Value=c2(3)
  c11 : Constant  Value=c2(2)
  c12 : Constant  Value=c2(1)
  yc3 : Outport
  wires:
  Vc2/1 -> Fcn/1, Product1/2
  Product1/1 -> Sum/2
  c10/1 -> Sum/3
  c12/1 -> Product/1
  Fcn/1 -> Product/2
  Product/1 -> Sum/1
  c11/1 -> Product1/1
  Sum/1 -> yc3/1

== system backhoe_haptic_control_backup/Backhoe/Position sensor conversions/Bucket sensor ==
  Vc4 : Inport
  Fcn : Fcn  Expr=u^2
  Product : Product
  Product1 : Product
  Sum : Sum  Inputs=+++
  c10 : Constant  Value=c4(3)
  c11 : Constant  Value=c4(2)
  c12 : Constant  Value=c4(1)
  yc5 : Outport
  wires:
  Vc4/1 -> Fcn/1, Product1/2
  Product1/1 -> Sum/2
  c10/1 -> Sum/3
  c12/1 -> Product/1
  Fcn/1 -> Product/2
  Product/1 -> Sum/1
  c11/1 -> Product1/1
  Sum/1 -> yc5/1

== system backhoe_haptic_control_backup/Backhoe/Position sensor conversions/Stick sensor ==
  Vc3 : Inport
  Fcn : Fcn  Expr=u^2
  Product : Product
  Product1 : Product
  Sum : Sum  Inputs=+++
  c10 : Constant  Value=c3(3)
  c11 : Constant  Value=c3(2)
  c12 : Constant  Value=c3(1)
  yc4 : Outport
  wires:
  Vc3/1 -> Fcn/1, Product1/2
  Product1/1 -> Sum/2
  c10/1 -> Sum/3
  c12/1 -> Product/1
  Fcn/1 -> Product/2
  Product/1 -> Sum/1
  c11/1 -> Product1/1
  Sum/1 -> yc4/1

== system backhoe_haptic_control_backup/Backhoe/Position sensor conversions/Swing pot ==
  Vc1 : Inport
  Fcn : Fcn  Expr=u^2
  Product : Product
  Product1 : Product
  Sum : Sum  Inputs=+++
  c10 : Constant  Value=c1(3)
  c11 : Constant  Value=c1(2)
  c12 : Constant  Value=c1(1)
  q1 : Outport
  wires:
  Vc1/1 -> Fcn/1, Product1/2
  Product1/1 -> Sum/2
  c10/1 -> Sum/3
  c12/1 -> Product/1
  Fcn/1 -> Product/2
  Product/1 -> Sum/1
  c11/1 -> Product1/1
  Sum/1 -> q1/1

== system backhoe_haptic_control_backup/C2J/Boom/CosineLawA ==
  r1 : Inport
  r2 : Inport  Port=2
  r3 : Inport  Port=3
  Fcn1 : Fcn  Expr=u^2
  Fcn2 : Fcn  Expr=u^2
  Fcn3 : Fcn  Expr=u^2
  Gain : Gain  Gain=2
  Product : Product
  Product1 : Product  Inputs=*/
  Sum : Sum  Inputs=++-
  Trigonometric Function : Trigonometry  Operator=acos
  theta : Outport
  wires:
  r3/1 -> Fcn3/1
  Fcn1/1 -> Sum/1
  Fcn2/1 -> Sum/2
  Fcn3/1 -> Sum/3
  r2/1 -> Fcn2/1, Product/1
  r1/1 -> Fcn1/1, Product/2
  Product/1 -> Gain/1
  Sum/1 -> Product1/1
  Gain/1 -> Product1/2
  Product1/1 -> Trigonometric Function/1
  Trigonometric Function/1 -> theta/1

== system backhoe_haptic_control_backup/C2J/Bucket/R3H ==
  THF3 : Inport
  RFH : Inport  Port=2
  Constant : Constant  Value=2
  Product : Product  Inputs=4
  R3F : Constant  Value=R3F
  Sum2 : Sum  Inputs=-++
  cosine : Trigonometry  Operator=cos
  sqr : Fcn  Expr=u^2
  sqr1 : Fcn  Expr=u^2
  sqrt : Fcn  Expr=sqrt(u)
  R3H : Outport
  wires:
  R3F/1 -> sqr/1, Product/2
  sqr1/1 -> Sum2/3
  Constant/1 -> Product/1
  [RFH] -> Product/3
  sqr/1 -> Sum2/2
  Product/1 -> Sum2/1
  cosine/1 -> Product/4
  Sum2/1 -> sqrt/1
  THF3/1 -> cosine/1
  sqrt/1 -> R3H/1
  RFH/1 -> sqr1/1, [RFH]

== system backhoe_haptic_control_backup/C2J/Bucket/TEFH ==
  r1 : Inport
  r2 : Inport  Port=2
  r3 : Inport  Port=3
  Fcn1 : Fcn  Expr=u^2
  Fcn2 : Fcn  Expr=u^2
  Fcn3 : Fcn  Expr=u^2
  Gain : Gain  Gain=2
  Product : Product
  Product1 : Product  Inputs=*/
  Sum : Sum  Inputs=++-
  Trigonometric Function : Trigonometry  Operator=acos
  TEFH : Outport
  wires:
  r3/1 -> Fcn3/1
  Fcn1/1 -> Sum/1
  Fcn2/1 -> Sum/2
  Fcn3/1 -> Sum/3
  r2/1 -> Fcn2/1, Product/1
  r1/1 -> Fcn1/1, Product/2
  Product/1 -> Gain/1
  Sum/1 -> Product1/1
  Gain/1 -> Product1/2
  Product1/1 -> Trigonometric Function/1
  Trigonometric Function/1 -> TEFH/1

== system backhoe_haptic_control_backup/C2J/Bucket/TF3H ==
  r1 : Inport
  r2 : Inport  Port=2
  r3 : Inport  Port=3
  Fcn1 : Fcn  Expr=u^2
  Fcn2 : Fcn  Expr=u^2
  Fcn3 : Fcn  Expr=u^2
  Gain : Gain  Gain=2
  Product : Product
  Product1 : Product  Inputs=*/
  Sum : Sum  Inputs=++-
  Trigonometric Function : Trigonometry  Operator=acos
  TF3H : Outport
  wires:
  r3/1 -> Fcn3/1
  Fcn1/1 -> Sum/1
  Fcn2/1 -> Sum/2
  Fcn3/1 -> Sum/3
  r2/1 -> Fcn2/1, Product/1
  r1/1 -> Fcn1/1, Product/2
  Product/1 -> Gain/1
  Sum/1 -> Product1/1
  Gain/1 -> Product1/2
  Product1/1 -> Trigonometric Function/1
  Trigonometric Function/1 -> TF3H/1

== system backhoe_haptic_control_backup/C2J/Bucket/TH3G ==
  r1 : Inport
  r2 : Inport  Port=2
  r3 : Inport  Port=3
  Fcn1 : Fcn  Expr=u^2
  Fcn2 : Fcn  Expr=u^2
  Fcn3 : Fcn  Expr=u^2
  Gain : Gain  Gain=2
  Product : Product
  Product1 : Product  Inputs=*/
  Sum : Sum  Inputs=++-
  Trigonometric Function : Trigonometry  Operator=acos
  TH3G : Outport
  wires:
  r3/1 -> Fcn3/1
  Fcn1/1 -> Sum/1
  Fcn2/1 -> Sum/2
  Fcn3/1 -> Sum/3
  r2/1 -> Fcn2/1, Product/1
  r1/1 -> Fcn1/1, Product/2
  Product/1 -> Gain/1
  Sum/1 -> Product1/1
  Gain/1 -> Product1/2
  Product1/1 -> Trigonometric Function/1
  Trigonometric Function/1 -> TH3G/1

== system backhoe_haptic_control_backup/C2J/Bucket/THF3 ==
  TEFH : Inport
  Sum1 : Sum  Inputs=+--
  TDFE : Constant  Value=TDFE
  pi1 : Constant  Value=pi
  THF3 : Outport
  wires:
  pi1/1 -> Sum1/1
  TDFE/1 -> Sum1/2
  Sum1/1 -> THF3/1
  TEFH/1 -> Sum1/3

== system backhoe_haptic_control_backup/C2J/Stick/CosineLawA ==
  r1 : Inport
  r2 : Inport  Port=2
  r3 : Inport  Port=3
  Fcn1 : Fcn  Expr=u^2
  Fcn2 : Fcn  Expr=u^2
  Fcn3 : Fcn  Expr=u^2
  Gain : Gain  Gain=2
  Product : Product
  Product1 : Product  Inputs=*/
  Sum : Sum  Inputs=++-
  Trigonometric Function : Trigonometry  Operator=acos
  theta : Outport
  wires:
  r3/1 -> Fcn3/1
  Fcn1/1 -> Sum/1
  Fcn2/1 -> Sum/2
  Fcn3/1 -> Sum/3
  r2/1 -> Fcn2/1, Product/1
  r1/1 -> Fcn1/1, Product/2
  Product/1 -> Gain/1
  Sum/1 -> Product1/1
  Gain/1 -> Product1/2
  Product1/1 -> Trigonometric Function/1
  Trigonometric Function/1 -> theta/1

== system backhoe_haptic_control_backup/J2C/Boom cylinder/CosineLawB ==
  TA1B : Inport
  Constant : Constant  Value=2
  Product : Product  Inputs=4
  Sum2 : Sum  Inputs=-++
  cosine : Trigonometry  Operator=cos
  rA : Constant  Value=R1A
  rB : Constant  Value=R1B
  sqr : Fcn  Expr=u^2
  sqr1 : Fcn  Expr=u^2
  sqrt : Fcn  Expr=sqrt(u)
  yc3 : Outport
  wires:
  rA/1 -> sqr/1, Product/2
  sqr1/1 -> Sum2/3
  Constant/1 -> Product/1
  [rB] -> Product/3
  sqr/1 -> Sum2/2
  Product/1 -> Sum2/1
  cosine/1 -> Product/4
  Sum2/1 -> sqrt/1
  TA1B/1 -> cosine/1
  sqrt/1 -> yc3/1
  rB/1 -> sqr1/1, [rB]

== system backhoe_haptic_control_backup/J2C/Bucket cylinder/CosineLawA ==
  r1 : Inport
  r2 : Inport  Port=2
  r3 : Inport  Port=3
  Fcn1 : Fcn  Expr=u^2
  Fcn2 : Fcn  Expr=u^2
  Fcn3 : Fcn  Expr=u^2
  Gain : Gain  Gain=2
  Product : Product
  Product1 : Product  Inputs=*/
  Sum : Sum  Inputs=++-
  Trigonometric Function : Trigonometry  Operator=acos
  T3FG : Outport
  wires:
  r3/1 -> Fcn3/1
  Fcn1/1 -> Sum/1
  Fcn2/1 -> Sum/2
  Fcn3/1 -> Sum/3
  r2/1 -> Fcn2/1, Product/1
  r1/1 -> Fcn1/1, Product/2
  Product/1 -> Gain/1
  Sum/1 -> Product1/1
  Gain/1 -> Product1/2
  Product1/1 -> Trigonometric Function/1
  Trigonometric Function/1 -> T3FG/1

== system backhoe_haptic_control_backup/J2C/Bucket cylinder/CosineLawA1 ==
  r1 : Inport
  r2 : Inport  Port=2
  r3 : Inport  Port=3
  Fcn1 : Fcn  Expr=u^2
  Fcn2 : Fcn  Expr=u^2
  Fcn3 : Fcn  Expr=u^2
  Gain : Gain  Gain=2
  Product : Product
  Product1 : Product  Inputs=*/
  Sum : Sum  Inputs=++-
  Trigonometric Function : Trigonometry  Operator=acos
  THFG : Outport
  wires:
  r3/1 -> Fcn3/1
  Fcn1/1 -> Sum/1
  Fcn2/1 -> Sum/2
  Fcn3/1 -> Sum/3
  r2/1 -> Fcn2/1, Product/1
  r1/1 -> Fcn1/1, Product/2
  Product/1 -> Gain/1
  Sum/1 -> Product1/1
  Gain/1 -> Product1/2
  Product1/1 -> Trigonometric Function/1
  Trigonometric Function/1 -> THFG/1

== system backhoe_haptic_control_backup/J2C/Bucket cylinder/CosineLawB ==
  TG3F : Inport
  Constant : Constant  Value=2
  Product : Product  Inputs=4
  Sum2 : Sum  Inputs=-++
  cosine : Trigonometry  Operator=cos
  rA : Constant  Value=R3F
  rB : Constant  Value=R3G
  sqr : Fcn  Expr=u^2
  sqr1 : Fcn  Expr=u^2
  sqrt : Fcn  Expr=sqrt(u)
  rFG : Outport
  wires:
  rA/1 -> sqr/1, Product/2
  sqr1/1 -> Sum2/3
  Constant/1 -> Product/1
  [rB] -> Product/3
  sqr/1 -> Sum2/2
  Product/1 -> Sum2/1
  cosine/1 -> Product/4
  Sum2/1 -> sqrt/1
  TG3F/1 -> cosine/1
  sqrt/1 -> rFG/1
  rB/1 -> sqr1/1, [rB]

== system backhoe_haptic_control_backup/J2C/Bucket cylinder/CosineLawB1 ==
  TEFH : Inport
  Constant : Constant  Value=2
  Product : Product  Inputs=4
  Sum2 : Sum  Inputs=-++
  cosine : Trigonometry  Operator=cos
  rA : Constant  Value=REF
  rB : Constant  Value=RFH
  sqr : Fcn  Expr=u^2
  sqr1 : Fcn  Expr=u^2
  sqrt : Fcn  Expr=sqrt(u)
  yc5 : Outport
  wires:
  rA/1 -> sqr/1, Product/2
  sqr1/1 -> Sum2/3
  Constant/1 -> Product/1
  [rB] -> Product/3
  sqr/1 -> Sum2/2
  Product/1 -> Sum2/1
  cosine/1 -> Product/4
  Sum2/1 -> sqrt/1
  TEFH/1 -> cosine/1
  sqrt/1 -> yc5/1
  rB/1 -> sqr1/1, [rB]

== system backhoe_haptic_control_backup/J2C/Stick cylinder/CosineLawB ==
  TC2D : Inport
  Constant : Constant  Value=2
  Product : Product  Inputs=4
  Sum2 : Sum  Inputs=-++
  cosine : Trigonometry  Operator=cos
  rA : Constant  Value=R2C
  rB : Constant  Value=R2D
  sqr : Fcn  Expr=u^2
  sqr1 : Fcn  Expr=u^2
  sqrt : Fcn  Expr=sqrt(u)
  yc4 : Outport
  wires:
  rA/1 -> sqr/1, Product/2
  sqr1/1 -> Sum2/3
  Constant/1 -> Product/1
  [rB] -> Product/3
  sqr/1 -> Sum2/2
  Product/1 -> Sum2/1
  cosine/1 -> Product/4
  Sum2/1 -> sqrt/1
  TC2D/1 -> cosine/1
  sqrt/1 -> yc4/1
  rB/1 -> sqr1/1, [rB]

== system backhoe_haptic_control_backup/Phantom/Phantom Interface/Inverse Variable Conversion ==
  doubles : Inport
  uint32s : Inport  Port=2
  Constant : Constant
  Demux : Demux
  Demux1 : Demux
  Demux2 : Demux  Outputs=2
  Homogenious Coordinate Transformation : Gain  Gain=com.Ph2Bh_Transform  Multiplication=Matrix(K*u)  ShowAdditionalParam=on
  Mux : Mux
  Mux1 : Mux
  Terminator : Terminator
  Yp : Outport
  Ph_Time : Outport  Port=2
  Ph_Flag : Outport  Port=3
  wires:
  doubles/1 -> Demux/1
  Demux/1 -> Mux/1  "xp"
  Demux/2 -> Mux/2  "yp"
  Demux/3 -> Mux/3  "zp"
  Mux/1 -> Homogenious Coordinate Transformation/1
  Demux2/1 -> Ph_Time/1
  Demux2/2 -> Ph_Flag/1
  Demux/4 -> [Bucket]
  Constant/1 -> Mux/4
  Homogenious Coordinate Transformation/1 -> Demux1/1
  Demux1/4 -> Terminator/1
  Mux1/1 -> Yp/1
  Demux1/3 -> Mux1/3
  Demux1/2 -> Mux1/2
  Demux1/1 -> Mux1/1
  [Bucket] -> Mux1/4
  uint32s/1 -> Demux2/1

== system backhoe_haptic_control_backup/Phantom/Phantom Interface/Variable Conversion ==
  note: Sends time in milliseconds (unit32)
  note: Sends flag as unit32
  note: Position variable are doubles
  note: Notes: Yb = the vector describing the backhoe (x,y,x and bucket anlge)
  note: xb,yb,zb are the coornates of the backhoe tip position transformed into Phantom coordinates
  Yb : Inport
  Bh_Time : Inport  Port=2
  Bh_Flag : Inport  Port=3
  Constant : Constant
  Demux : Demux
  Demux1 : Demux
  Homogenious Coordinate Transformation : Gain  Gain=com.Bh2Ph_Transform  Multiplication=Matrix(K*u)  ShowAdditionalParam=on
  Mux : Mux
  Mux1 : Mux
  Mux2 : Mux  Inputs=2
  Terminator1 : Terminator
  doubles : Outport
  uint32s : Outport  Port=2
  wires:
  Demux/1 -> Mux/1
  Demux/2 -> Mux/2
  Yb/1 -> Demux/1
  Demux/3 -> Mux/3
  Bh_Flag/1 -> Mux2/2
  Constant/1 -> Mux/4
  Homogenious Coordinate Transformation/1 -> Demux1/1
  Mux/1 -> Homogenious Coordinate Transformation/1
  Demux1/1 -> Mux1/1  "xb"
  Demux1/2 -> Mux1/2  "yb"
  Demux1/3 -> Mux1/3  "zb"
  Demux1/4 -> Terminator1/1
  Bh_Time/1 -> Mux2/1
  Mux2/1 -> uint32s/1
  Mux1/1 -> doubles/1
  Demux/4 -> Mux1/4

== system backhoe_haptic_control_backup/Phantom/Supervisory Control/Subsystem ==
  Yp : Inport
  Constant : Constant  Value=0
  Constant1 : Constant  Value=pi/3
  Demux : Demux
  Mux : Mux  Inputs=6
  Selector : Selector  Elements=[1 2 3 4]  InputPortWidth=6
  Y_Bh_REF : Outport
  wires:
  Mux/1 -> Selector/1
  Selector/1 -> Y_Bh_REF/1
  Yp/1 -> Demux/1
  Demux/1 -> Mux/1
  Demux/4 -> Mux/4
  Demux/3 -> Mux/3
  Demux/2 -> Mux/2
  Constant/1 -> Mux/5
  Constant1/1 -> Mux/6

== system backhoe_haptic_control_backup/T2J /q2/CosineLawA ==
  r1 : Inport
  r2 : Inport  Port=2
  r3 : Inport  Port=3
  Fcn1 : Fcn  Expr=u^2
  Fcn2 : Fcn  Expr=u^2
  Fcn3 : Fcn  Expr=u^2
  Gain : Gain  Gain=2
  Product : Product
  Product1 : Product  Inputs=*/
  Sum : Sum  Inputs=++-
  Trigonometric Function : Trigonometry  Operator=acos
  theta : Outport
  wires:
  r3/1 -> Fcn3/1
  Fcn1/1 -> Sum/1
  Fcn2/1 -> Sum/2
  Fcn3/1 -> Sum/3
  r2/1 -> Fcn2/1, Product/1
  r1/1 -> Fcn1/1, Product/2
  Product/1 -> Gain/1
  Sum/1 -> Product1/1
  Gain/1 -> Product1/2
  Product1/1 -> Trigonometric Function/1
  Trigonometric Function/1 -> theta/1

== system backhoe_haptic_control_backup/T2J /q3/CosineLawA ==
  r1 : Inport
  r2 : Inport  Port=2
  r3 : Inport  Port=3
  Fcn1 : Fcn  Expr=u^2
  Fcn2 : Fcn  Expr=u^2
  Fcn3 : Fcn  Expr=u^2
  Gain : Gain  Gain=2
  Product : Product
  Product1 : Product  Inputs=*/
  Sum : Sum  Inputs=++-
  Trigonometric Function : Trigonometry  Operator=acos
  theta : Outport
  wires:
  r3/1 -> Fcn3/1
  Fcn1/1 -> Sum/1
  Fcn2/1 -> Sum/2
  Fcn3/1 -> Sum/3
  r2/1 -> Fcn2/1, Product/1
  r1/1 -> Fcn1/1, Product/2
  Product/1 -> Gain/1
  Sum/1 -> Product1/1
  Gain/1 -> Product1/2
  Product1/1 -> Trigonometric Function/1
  Trigonometric Function/1 -> theta/1

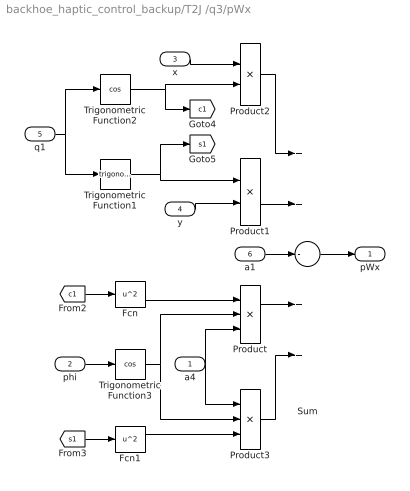
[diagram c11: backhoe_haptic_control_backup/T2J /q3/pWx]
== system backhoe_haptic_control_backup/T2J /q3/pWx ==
  a4 : Inport
  phi : Inport  Port=2
  x : Inport  Port=3
  y : Inport  Port=4
  q1 : Inport  Port=5
  a1 : Inport  Port=6
  Fcn : Fcn  Expr=u^2
  Fcn1 : Fcn  Expr=u^2
  Product : Product  Inputs=3
  Product1 : Product
  Product2 : Product
  Product3 : Product  Inputs=3
  Sum : Sum  Inputs=++-++
  Trigonometric Function1 : Trigonometry
  Trigonometric Function2 : Trigonometry  Operator=cos
  Trigonometric Function3 : Trigonometry  Operator=cos
  pWx : Outport
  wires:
  Product2/1 -> Sum/1
  Product1/1 -> Sum/2
  x/1 -> Product2/1
  Sum/1 -> pWx/1
  a1/1 -> Sum/3
  q1/1 -> Trigonometric Function2/1, Trigonometric Function1/1
  y/1 -> Product1/2
  Trigonometric Function1/1 -> Product1/1, [s1]
  Trigonometric Function2/1 -> Product2/2, [c1]
  Product/1 -> Sum/4
  Product3/1 -> Sum/5
  [c1] -> Fcn/1
  Fcn/1 -> Product/1
  a4/1 -> Product/3, Product3/1
  Trigonometric Function3/1 -> Product/2, Product3/2
  Fcn1/1 -> Product3/3
  [s1] -> Fcn1/1
  phi/1 -> Trigonometric Function3/1

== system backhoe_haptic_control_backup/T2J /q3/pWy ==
  z : Inport
  phi : Inport  Port=2
  a4 : Inport  Port=3
  Product : Product
  Sum : Sum  Inputs=|++
  Trigonometric Function : Trigonometry
  pWy : Outport
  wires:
  Trigonometric Function/1 -> Product/2
  a4/1 -> Product/1
  Product/1 -> Sum/1
  Sum/1 -> pWy/1
  phi/1 -> Trigonometric Function/1
  z/1 -> Sum/2
